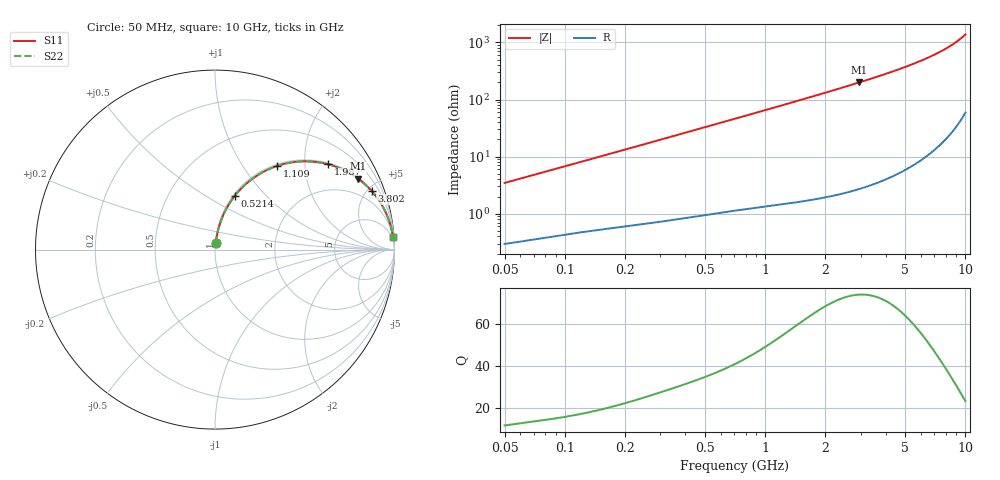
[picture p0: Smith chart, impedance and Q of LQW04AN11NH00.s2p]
!Murata Part Number: LQW04AN11NH00
!These Parameters are Measured in Series Mode Connection
!  o--[Z]--o
!Port1  Port2
!  o-------o
!Freq. Start=50[MHz] Stop=10[GHz], 401[Steps]
# Hz S RI R 50
!Freq.(Hz)	S 11(Real)	S 11(Imag)	S 21(Real)	S 21(Imag)	S 12(Real)	S 12(Imag)	S 22(Real)	S 22(Imag)
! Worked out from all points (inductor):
!   401 points, 50 MHz to 10 GHz, reference 50 ohm
!   read as one part in series: L = 10.9 nH near 51.34 MHz
!   highest Q = 73.7 at 2.956 GHz (marker M1), where L = 10.8 nH
!   S11 on the Smith chart (normalised r, x): 50 MHz: 1.01, +0.07; 521.4 MHz: 1.02, +0.68; 1.109 GHz: 1.03, +1.45; 1.987 GHz: 1.04, +2.62; 3.802 GHz: 1.07, +5.31; 10 GHz: 2, +28
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5e7  0.00413 0.0343  0.9959 -0.0343  0.9959 -0.0343  0.00413 0.0343
7.948957e7  0.00668 0.0536  0.9933 -0.0536  0.9933 -0.0536  0.00668 0.0536
1.214486e8  0.0113 0.0804  0.9887 -0.0804  0.9887 -0.0804  0.0113 0.0804
1.930779e8  0.0218 0.1249  0.9782 -0.1249  0.9782 -0.1249  0.0218 0.1249
2.949953e8  0.0429 0.185  0.9571 -0.185  0.9571 -0.185  0.0429 0.185
4.000592e8  0.0714 0.242  0.9286 -0.242  0.9286 -0.242  0.0714 0.242
5.214057e8  0.1112 0.3005  0.8888 -0.3005  0.8888 -0.3005  0.1112 0.3005
7.071068e8  0.1817 0.3735  0.8183 -0.3735  0.8183 -0.3735  0.1817 0.3735
8.85684e8  0.2549 0.425  0.7451 -0.425  0.7451 -0.425  0.2549 0.425
1.10936e9  0.3466 0.4663  0.6534 -0.4663  0.6534 -0.4663  0.3466 0.4663
1.389525e9  0.453 0.4893  0.547 -0.4893  0.547 -0.4893  0.453 0.4893
1.717543e9  0.5589 0.4888  0.4411 -0.4888  0.4411 -0.4888  0.5589 0.4888
1.986945e9  0.6303 0.4754  0.3697 -0.4754  0.3697 -0.4754  0.6303 0.4754
2.391784e9  0.7145 0.4448  0.2855 -0.4448  0.2855 -0.4448  0.7145 0.4448
2.956399e9  0.7968 0.3956  0.2032 -0.3956  0.2032 -0.3956  0.7968 0.3956
3.802437e9  0.8725 0.3267  0.1275 -0.3267  0.1275 -0.3267  0.8725 0.3267
4.171863e9  0.8944 0.3002  0.1056 -0.3002  0.1056 -0.3002  0.8944 0.3002
5.509778e9  0.9439 0.2218  0.0561 -0.2218  0.0561 -0.2218  0.9439 0.2218
6.993273e9  0.9706 0.1586  0.0294 -0.1586  0.0294 -0.1586  0.9706 0.1586
7.672705e9  0.978 0.1352  0.022 -0.1352  0.022 -0.1352  0.978 0.1352
8.418147e9  0.9839 0.1124  0.0161 -0.1124  0.0161 -0.1124  0.9839 0.1124
1e10  0.9918 0.0715  0.00825 -0.0715  0.00825 -0.0715  0.9918 0.0715
